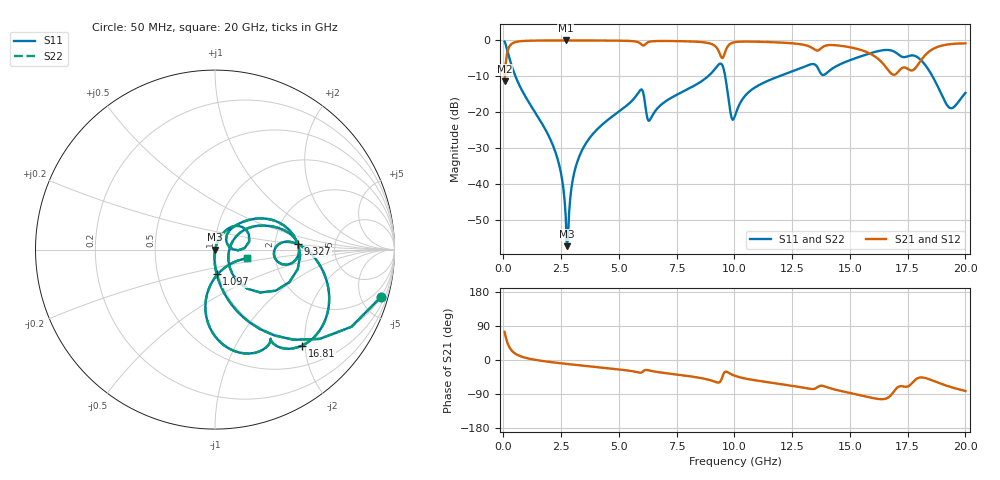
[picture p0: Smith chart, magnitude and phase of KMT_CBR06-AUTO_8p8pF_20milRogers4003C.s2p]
! Data measured by Modelithics Inc. support@modelithics.com 813-866-6335
! KEMET CBR06-AUTO 8.8pF, Pad Width= 0.851mm, Pad Length= 0.64mm, Pad Gap= 0.62mm, 20mil Rogers 4003C substrate Data, January 2022
# hz S ma R 50
! 2 Port Network Data from SP1.SP block
! freq  magS11  angS11  magS21  angS21  magS12  angS12  magS22  angS22
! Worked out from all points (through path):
!   401 points, 50 MHz to 20 GHz, reference 50 ohm
!   highest |S21| = -0.01 dB at 2.693 GHz (marker M1); lowest = -11.4 dB at 50 MHz (marker M2)
!   group delay of S21, straight-line fit = 13.3 ps
!   lowest |S11| = -57.4 dB at 2.743 GHz (marker M3), VSWR 1.00, Z = 50.1 - j0.115 ohm
!   |S11| at or under -10 dB: 520.6 MHz to 8.858 GHz (8.337 GHz wide, 178 % of centre); 9.599 GHz to 11.93 GHz (2.333 GHz wide, 21.7 % of centre); 18.57 GHz to end of sweep
!   |S22| runs from -57.4 to -0.3 dB; largest |S21 - S12| = 0
!   S11 on the Smith chart (normalised r, x): 50 MHz: 0.98, -7.10; 1.097 GHz: 0.98, -0.27; 9.327 GHz: 2.71, +0.21; 16.81 GHz: 0.87, -1.94; 20 GHz: 1.43, -0.15
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5e7  0.9633 -15.8  0.2683 74.2  0.2683 74.2  0.9633 -15.8
3.99125e8  0.4033 -67.7  0.9145 22.3  0.9145 22.3  0.4033 -67.7
1.097375e9  0.1375 -86.0  0.9898 3.7  0.9898 3.7  0.1375 -86.0
2.294375e9  0.02513 -95.4  0.9988 -7.3  0.9988 -7.3  0.02513 -95.4
2.693375e9  0.003613 -85.6  0.999 -10.1  0.999 -10.1  0.003613 -85.6
2.74325e9  0.001354 -58.1  0.999 -10.4  0.999 -10.4  0.001354 -58.1
3.0425e9  0.01334 73.5  0.9988 -12.4  0.9988 -12.4  0.01334 73.5
3.391625e9  0.02897 73.4  0.9984 -14.6  0.9984 -14.6  0.02897 73.4
5.93525e9  0.2049 33.5  0.9013 -33.4  0.9013 -33.4  0.2049 33.5
6.284375e9  0.07571 23.4  0.95 -27.2  0.95 -27.2  0.07571 23.4
6.73325e9  0.1192 52.4  0.9818 -32.3  0.9818 -32.3  0.1192 52.4
9.32675e9  0.464 3.8  0.7011 -59.5  0.7011 -59.5  0.464 3.8
9.576125e9  0.3482 -43.4  0.656 -32.0  0.656 -32.0  0.3482 -43.4
1.0025e10  0.08909 13.8  0.9466 -41.8  0.9466 -41.8  0.08909 13.8
1.087288e10  0.2193 32.9  0.9609 -53.3  0.9609 -53.3  0.2193 32.9
1.336662e10  0.4683 0.8  0.7872 -76.7  0.7872 -76.7  0.4683 0.8
1.511225e10  0.5464 -3.6  0.7896 -88.5  0.7896 -88.5  0.5464 -3.6
1.670825e10  0.7336 -43.8  0.3681 -96.8  0.3681 -96.8  0.7336 -43.8
1.6808e10  0.7218 -47.9  0.3411 -90.6  0.3411 -90.6  0.7218 -47.9
1.845388e10  0.3682 -97.8  0.7096 -51.3  0.7096 -51.3  0.3682 -97.8
1.930175e10  0.1159 -65.5  0.8838 -70.1  0.8838 -70.1  0.1159 -65.5
2e10  0.1855 -15.4  0.9099 -81.6  0.9099 -81.6  0.1855 -15.4
